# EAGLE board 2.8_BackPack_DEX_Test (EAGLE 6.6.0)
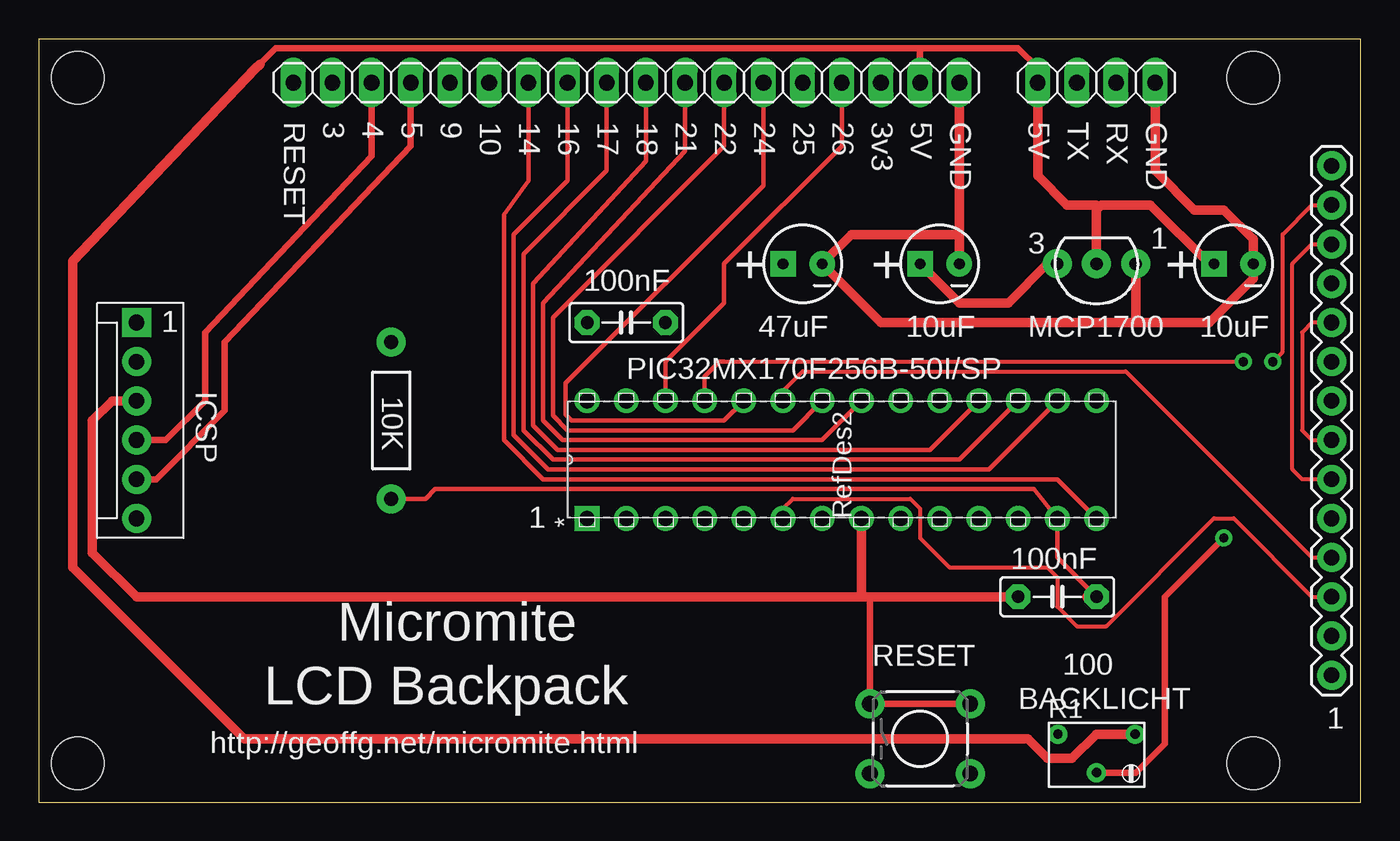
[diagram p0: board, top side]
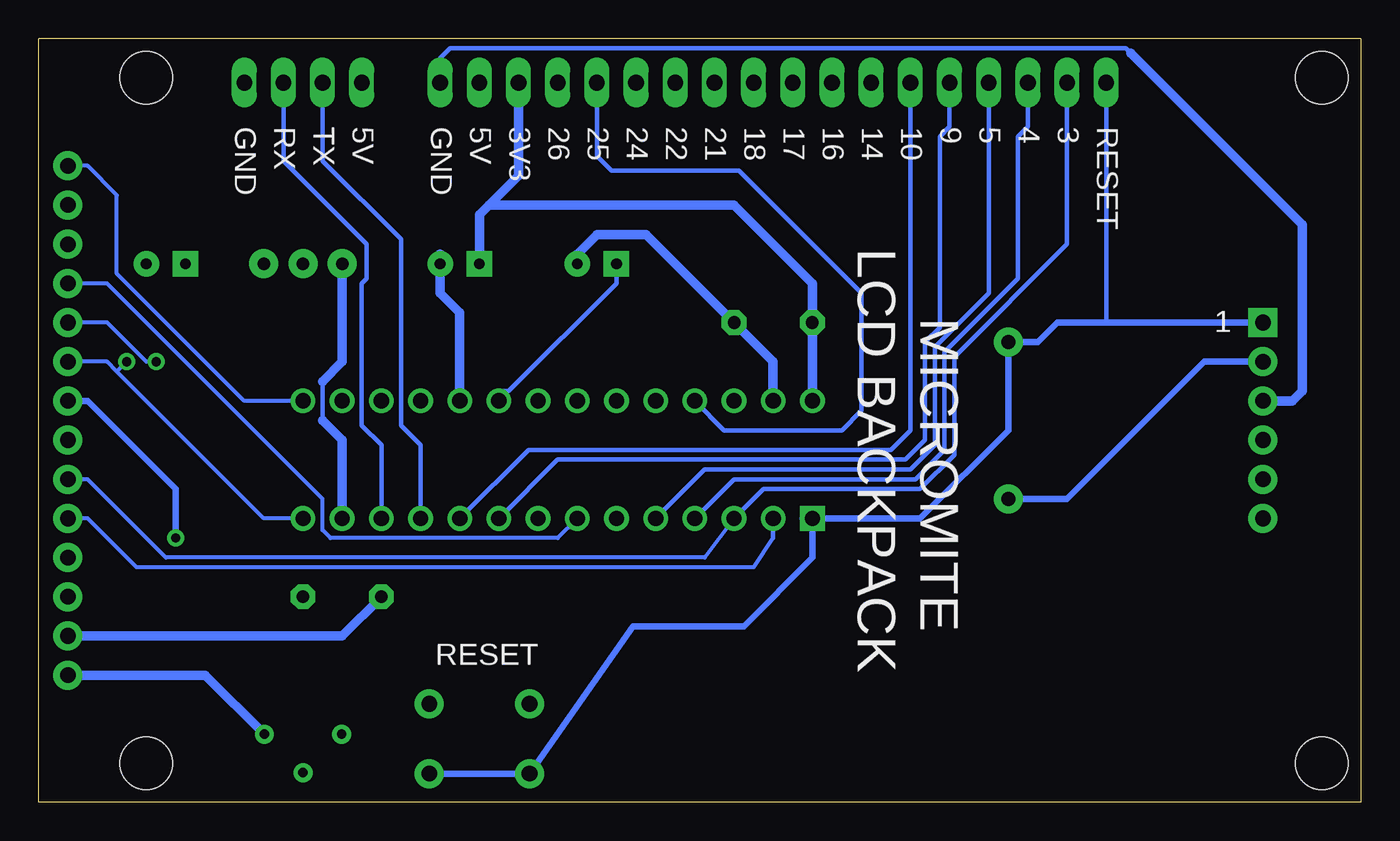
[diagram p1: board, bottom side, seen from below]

Size 85.72 x 49.53 mm. Coordinates in mm from the lower left corner, seen from the top.
Outline: 85.72,0 85.72,49.53 0,49.53 0,0 85.72,0
Copper layers (1*16): Top 0.035mm / dielectric 1.5mm / Bottom 0.035mm
Design rules "SparkFun *": minimum track width 10mil, minimum drill 20mil, track to track 8mil, track to pad 8mil, pad to pad 8mil, via to via 8mil, smd to smd 8mil, copper to edge 8mil, drill to drill 8mil, minimum pad ring 12mil, minimum via ring 10mil, stop-mask expansion 4mil, vias tented up to drill 25mil, thermal gap 10mil
Holes 3.4 mm at 2.54,2.54 2.54,46.99 78.74,2.54 78.74,46.99
tKeepout: area -1.1,43.4 to 6.1,50.6; area 75,43.4 to 82.2,50.6; area 75,-1.1 to 82.2,6.1; area -1.1,-1.1 to 6.1,6.1
bKeepout: area -1.1,43.4 to 6.1,50.6; area -1.1,-1.1 to 6.1,6.1; area 75,-1.1 to 82.2,6.1; area 75,43.4 to 82.2,50.6

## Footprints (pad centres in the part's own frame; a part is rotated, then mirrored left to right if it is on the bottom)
CPOL-RADIAL-10UF-25V = drill 0.7 pad 1.651 square: 1 1.27,0 | drill 0.7 pad 1.651: 2 -1.27,0
C5B2.5 = drill 0.813 pad 1.6 octagon: 1 -2.54,0; 2 2.54,0
1X14 = drill 1.016 pad 1.88: 1 0,0; 2 2.54,0; 3 5.08,0; 4 7.62,0; 5 10.16,0; 6 12.7,0; 7 15.24,0; 8 17.78,0; 9 20.32,0; 10 22.86,0; 11 25.4,0; 12 27.94,0; 13 30.48,0; 14 33.02,0
MOLEX-1X6 = drill 1.016 pad 1.88 square: 1 0,0 | drill 1.016 pad 1.88: 2 2.54,0; 3 5.08,0; 4 7.62,0; 5 10.16,0; 6 12.7,0
1X04 = drill 1.016 long: 1 -3.81,0; 2 -1.27,0; 3 1.27,0; 4 3.81,0
1X18 = drill 1.016 long: 1 -21.59,0; 2 -19.05,0; 3 -16.51,0; 4 -13.97,0; 5 -11.43,0; 6 -8.89,0; 7 -6.35,0; 8 -3.81,0; 9 -1.27,0; 10 1.27,0; 11 3.81,0; 12 6.35,0; 13 8.89,0; 14 11.43,0; 15 13.97,0; 16 16.51,0; 17 19.05,0; 18 21.59,0
TO-92-AMMO = drill 0.813 pad 1.88: 1 -2.54,0; 2 0,0; 3 2.54,0
RTRIM74W = drill 0.61: 1 -1.25,-2.5; 2 1.25,0; 3 -1.25,2.5
AXIAL-0.4 = drill 0.9 pad 1.88: P$1 -5.08,0; P$2 5.08,0
TACTILE-PTH = drill 1.016 pad 1.88: 1 -3.251,2.261; 2 3.251,2.261; 3 -3.251,-2.261; 4 3.251,-2.261
SPDIP28_300MC = drill 0.991 square: 1 -7.62,33.02 | drill 0.991: 2 -7.62,30.48; 3 -7.62,27.94; 4 -7.62,25.4; 5 -7.62,22.86; 6 -7.62,20.32; 7 -7.62,17.78; 8 -7.62,15.24; 9 -7.62,12.7; 10 -7.62,10.16; 11 -7.62,7.62; 12 -7.62,5.08; 13 -7.62,2.54; 14 -7.62,0; 15 0,0; 16 0,2.54; 17 0,5.08; 18 0,7.62; 19 0,10.16; 20 0,12.7; 21 0,15.24; 22 0,17.78; 23 0,20.32; 24 0,22.86; 25 0,25.4; 26 0,27.94; 27 0,30.48; 28 0,33.02

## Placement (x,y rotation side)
C1  [CPOL-RADIAL-10UF-25V]  49.53,34.92 180 top
C2  [CPOL-RADIAL-10UF-25V]  77.47,34.92 180 top
C3  [CPOL-RADIAL-10UF-25V]  58.42,34.92 180 top
C10  100nF  [C5B2.5]  66.04,13.34 0 top
C11  100nF  [C5B2.5]  38.1,31.11 180 top
JP1  M14  [1X14]  83.82,8.26 90 top
JP2  [MOLEX-1X6]  6.35,31.11 270 top
JP4  [1X04]  68.58,46.67 0 top
JP5  [1X18]  38.1,46.67 0 top
Q1  [TO-92-AMMO]  68.58,34.92 180 top
R1  [RTRIM74W]  68.58,3.17 270 top
R2  10K  [AXIAL-0.4]  22.86,24.77 270 top
S1  [TACTILE-PTH]  57.15,4.13 0 top
U2  [SPDIP28_300MC]  68.58,26.04 90 top

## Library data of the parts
C1-C3 JP1 JP2 Q1 R2 S1 = SparkFun
C10 C11 = capacitor-wima
JP4 JP5 = pinhead
R1 = resistor
U2 = Microchip-grg

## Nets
GND: C1.2 C2.2 C3.2 C10.1 C11.1 JP1.2 JP2.3 JP4.4 JP5.18 Q1.1 S1.1 S1.2 U2.8 U2.19 U2.27
N$1: C1.1 U2.20
N$2: JP2.1 JP5.1 R2.P$1 S1.3 S1.4 U2.1
N$3: JP1.14 U2.15
N$4: C2.1 JP1.1 JP4.1 JP5.17 Q1.2 R1.3
N$5: JP4.3 U2.12
N$6: JP4.2 U2.11
N$7: JP5.12 U2.22
N$8: JP1.5 U2.2
N$9: JP1.6 JP1.12 JP5.2 U2.3
N$10: JP1.4 U2.23
N$11: JP1.7 JP1.10 JP5.14 U2.25
N$12: JP1.8 R1.2
N$13: JP2.5 JP5.4 U2.5
N$14: JP1.11 U2.7
N$15: JP1.9 JP1.13 JP5.7 U2.14
N$17: JP1.3 U2.6
N$18: JP5.5 U2.9
N$19: JP5.6 U2.10
N$20: JP5.8 U2.16
N$21: JP5.9 U2.17
N$22: JP5.10 U2.18
N$23: JP5.11 U2.21
N$25: JP5.13 U2.24
N$26: JP5.15 U2.26
N$27: JP2.4 JP5.3 U2.4
VDD: C3.1 C10.2 C11.2 JP2.2 JP5.16 Q1.3 R2.P$2 U2.13 U2.28

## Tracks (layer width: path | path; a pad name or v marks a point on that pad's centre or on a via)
GND
  Top 0.406: 53.98,13.34 53.9,13.26 S1.1 S1.2
  Top 0.61: 61.59,13.34 C10.1 56.52,13.34 | 56.52,13.34 55.88,13.34 | 59.69,35.56 C3.2 59.69,36.83 | 53.34,13.34 53.98,13.34 56.52,13.34 | 53.34,13.34 U2.8 | 59.69,36.83 52.7,36.83 C1.2 54.61,31.11 71.12,31.11 | 71.12,31.11 75.88,31.11 78.74,33.97 C2.2 78.74,36.51 76.83,38.42 74.93,38.42 72.39,40.96 JP4.4 | 71.12,31.11 Q1.1 | 53.34,13.34 6.35,13.34 3.49,16.19 3.49,24.77 4.76,26.04 JP2.3 | 59.69,36.83 JP5.18
  Bottom 0.305: 14.92,48.58 15.24,48.9 59.05,48.9 59.69,48.26 JP5.18
  Bottom 0.61: C10.1 66.04,10.79 JP1.2 | U2.27 38.1,28.57 C11.1 46.35,36.83 49.53,36.83 50.8,35.56 C1.2 | 59.69,35.56 C3.2 59.69,33.02 58.42,31.75 U2.19 | JP2.3 4.45,26.04 3.81,26.67 3.81,37.47 14.92,48.58
N$1
  Bottom 0.305: C1.1 48.26,33.66 55.24,26.67 55.88,26.67 U2.20
N$2
  Bottom 0.305: 16.51,31.11 JP5.1
  Bottom 0.406: 35.56,17.78 35.56,15.88 40.01,11.43 47.19,11.43 S1.3 S1.4 | 35.56,17.78 U2.1 | 5.71,31.11 JP2.1 16.51,31.11 19.68,31.11 20.95,29.84 R2.P$1 22.86,24.13 28.57,18.41 36.2,18.41 35.56,17.78
N$3
  Bottom 0.254: U2.15 72.39,26.04 80.64,34.29 80.64,39.37 82.55,41.27 JP1.14
N$4
  Top 0.406: JP4.1 64.77,47.62 63.5,48.9 57.15,48.9 | 57.15,48.9 15.37,48.9 14.03,47.56 | 57.15,48.9 JP5.17
  Top 0.61: 68.58,38.42 68.58,38.73 66.67,38.73 64.77,40.64 JP4.1 | 68.58,38.42 Q1.2 | C2.1 75.88,34.92 72.07,38.73 68.9,38.73 68.58,38.42 | R1.3 68.56,4.42 66.99,2.86 65.41,2.86 64.14,4.13 13.34,4.13 2.22,15.24 2.22,35.12 14.03,47.56 14.35,47.88
  Bottom 0.61: JP1.1 74.91,8.26 R1.3
N$5
  Bottom 0.305: U2.12 63.5,23.18 64.77,24.45 64.77,33.66 64.45,33.97 64.45,36.2 69.85,41.59 JP4.3
N$6
  Bottom 0.305: U2.11 60.96,23.18 62.23,24.45 62.23,36.51 67.31,41.59 JP4.2
N$7
  Top 0.305: U2.22 48.9,24.13 34.29,24.13 33.34,25.08 33.34,31.43 44.45,42.55 JP5.12
N$8
  Bottom 0.254: 38.1,17.14 39.37,15.24 79.38,15.24 82.55,18.41 JP1.5
  Bottom 0.305: 38.1,17.14 U2.2
N$9
  Top 0.254: JP1.6 81.92,20.95 81.28,21.59 81.28,34.92 82.55,36.2 JP1.12
  Bottom 0.254: U2.3 42.55,15.88 77.47,15.88 82.55,20.95 JP1.6
  Bottom 0.305: U2.3 38.73,20.32 28.57,20.32 26.35,22.54 26.35,28.89 19.05,36.2 JP5.2
N$10
  Top 0.254: U2.23 48.26,26.67 49.53,27.94 70.48,27.94 82.55,15.88 JP1.4
N$11  (via drill 0.6)
  Top 0.254: 44.45,28.57 v78.11,28.57 | JP1.7 82.55,23.5 81.92,24.13 81.92,30.48 82.55,31.11 JP1.10
  Top 0.305: 44.45,28.57 44.13,28.57 43.18,27.62 U2.25
  Bottom 0.254: v78.11,28.57 78.74,28.57 81.28,31.11 JP1.10
  Bottom 0.305: U2.25 41.27,24.13 33.66,24.13 32.38,25.4 32.38,33.02 40.32,40.96 48.58,40.96 49.53,41.91 JP5.14
N$12  (via drill 0.6)
  Top 0.406: v76.83,17.14 73.03,13.34 73.03,3.81 71.12,1.91 68.6,1.91 R1.2
  Bottom 0.406: JP1.8 82.55,26.04 76.83,20.32 v76.83,17.14
N$13
  Top 0.406: JP5.4 24.13,42.55 12.06,29.84 12.06,25.4 7.62,20.95 JP2.5
  Bottom 0.305: U2.5 42.55,21.59 29.21,21.59 27.62,23.18 27.62,29.53 24.13,33.02 JP5.4
N$14
  Bottom 0.254: U2.7 52.07,17.14 66.8,17.14 67.31,17.65 67.31,19.68 81.28,33.66 JP1.11
N$15  (via drill 0.6)
  Top 0.254: JP1.13 82.55,38.73 80.64,36.83 80.64,29.21 v80.01,28.57
  Top 0.305: U2.14 66.04,20.95 32.7,20.95 30.16,23.5 30.16,38.1 31.75,40.32 JP5.7
  Bottom 0.254: U2.14 71.12,18.41 80.64,27.94 | 80.64,27.94 81.28,28.57 JP1.9 | 80.64,27.94 v80.01,28.57
N$17
  Top 0.254: U2.6 48.26,19.05 48.9,19.68 56.52,19.68 57.15,19.05 57.15,17.14 59.05,15.24 65.41,15.24 66.04,14.61 66.04,12.7 67.31,11.43 69.22,11.43 76.2,18.41 77.47,18.41 82.55,13.34 JP1.3 84.45,13.34
N$18
  Bottom 0.305: U2.9 52.07,22.23 29.53,22.23 28.26,23.5 28.26,29.84 27.3,30.8 27.3,43.18 26.67,43.81 JP5.5
N$19
  Bottom 0.305: U2.10 53.98,22.86 30.48,22.86 29.21,24.13 JP5.6
N$20
  Top 0.305: U2.16 61.59,21.59 33.02,21.59 30.8,23.81 30.8,36.83 34.29,40.32 JP5.8
N$21
  Top 0.305: U2.17 59.69,22.23 33.34,22.23 31.43,24.13 31.43,35.56 36.83,40.96 JP5.9
N$22
  Top 0.305: U2.18 57.78,22.86 33.66,22.86 32.07,24.45 32.07,33.66 39.37,41.59 JP5.10
N$23
  Top 0.305: U2.21 50.8,23.5 33.97,23.5 32.7,24.77 32.7,32.38 41.91,42.23 JP5.11
N$25
  Top 0.305: U2.24 44.45,24.77 34.54,24.77 34.16,25.15 34.16,27.18 46.99,40.01 JP5.13
N$26
  Top 0.305: U2.26 40.64,28.57 44.45,32.38 44.45,34.92 52.07,42.55 JP5.15
N$27
  Top 0.406: JP5.3 21.59,41.91 10.79,30.48 10.79,26.04 8.26,23.5 JP2.4
  Bottom 0.305: U2.4 40.64,20.95 28.89,20.95 26.99,22.86 26.99,29.21 22.23,33.97 22.23,43.18 21.59,43.81 JP5.3
VDD
  Top 0.305: C10.2 66.04,15.88 U2.13 64.52,20.32 25.72,20.32 25.08,19.68 R2.P$2
  Top 0.61: C10.2 67.94,13.34 | Q1.3 65.41,34.92 62.87,32.38 59.69,32.38 C3.1
  Bottom 0.305: 67.31,24.77 67.31,27.3
  Bottom 0.406: R2.P$2 19.05,19.68 10.16,28.57 JP2.2
  Bottom 0.61: U2.28 C11.2 35.56,33.66 40.64,38.73 56.52,38.73 | Q1.3 66.04,28.57 67.31,27.3 | U2.13 66.04,23.5 67.31,24.77 | C3.1 57.15,38.1 56.52,38.73 | 56.52,38.73 54.61,40.64 JP5.16

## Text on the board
tPlace: RESET | 3 | 4 | 5 | 9 | 10 | 14 | 16 | 17 | 18 | 21 | 22 | 24 | 25 | 26 | 3v3 | 5V | GND | 5V | TX | RX | GND | 3 | 1 | + | + | + | 100nF | 1 | 47uF | 10uF | MCP1700 | 10uF | ICSP | PIC32MX170F256B-50I/SP | 10K | 1 | 100nF | Micromite | RESET | 100 | LCD Backpack | BACKLICHT | 1 | http://geoffg.net/micromite.html
bPlace: RESET | 3 | 4 | 5 | 9 | 10 | 14 | 16 | 17 | 18 | 21 | 22 | 24 | 25 | 26 | 3V3 | 5V | GND | 5V | TX | RX | GND | LCD BACKPACK | MICROMITE | 1 | RESET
